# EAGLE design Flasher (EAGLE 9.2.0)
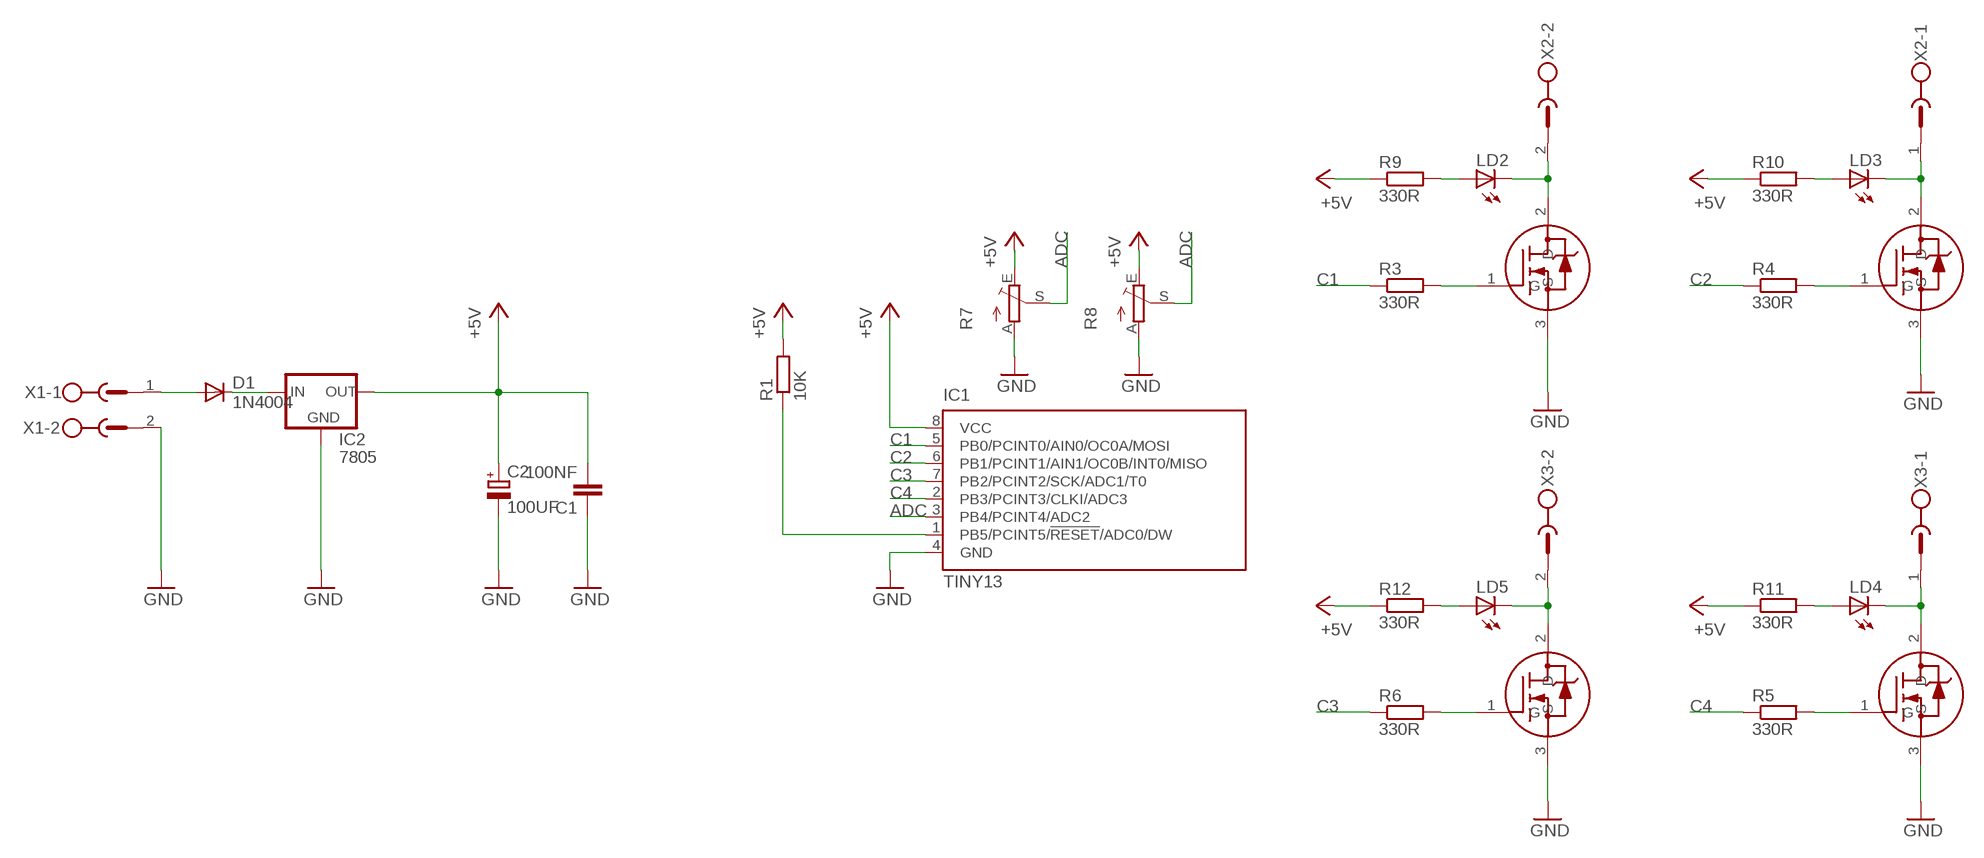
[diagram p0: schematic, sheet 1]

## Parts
C1  100NF  C-EU050-024X044  [C050-024X044]
C2  100UF  CPOL-EUE2.5-5  [E2,5-5]
D1  1N4004  [DO41-10]
IC1  TINY13  TINY13-20PU  [DIL08]
IC2  7805  78XXS  [78XXS]
LD2  LED5MM  [LED5MM]
LD3  LED5MM  [LED5MM]
LD4  LED5MM  [LED5MM]
LD5  LED5MM  [LED5MM]
R1  10K  R-EU_0204/7  [0204/7]
R3  330R  R-EU_0207/10  [0207/10]
R4  330R  R-EU_0207/10  [0207/10]
R5  330R  R-EU_0207/12  [0207/12]
R6  330R  R-EU_0207/10  [0207/10]
R7  TRIM_EU-B25U  [B25U]
R8  TRIM_EU-B25P  [B25P]
R9  330R  R-EU_0204/2V  [0204V]
R10  330R  R-EU_0204/2V  [0204V]
R11  330R  R-EU_0204/2V  [0204V]
R12  330R  R-EU_0204/2V  [0204V]
U$1  20N03  [DPAK]
U$2  20N03  [DPAK]
U$3  20N03  [DPAK]
U$4  20N03  [DPAK]
X1  MSTBV2  [MSTBV2]
X2  MSTBV2  [MSTBV2]
X3  MSTBV2  [MSTBV2]

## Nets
+5V: C1.2 C2.+ IC1.8(VCC) IC2.OUT R1.2 R7.E R8.E R9.1 R10.1 R11.1 R12.1
ADC: IC1.3(PB4/PCINT4/ADC2) R7.S R8.S
C1: IC1.5(PB0/PCINT0/AIN0/OC0A/MOSI) R3.1
C2: IC1.6(PB1/PCINT1/AIN1/OC0B/INT0/MISO) R4.1
C3: IC1.7(PB2/PCINT2/SCK/ADC1/T0) R6.1
C4: IC1.2(PB3/PCINT3/CLKI/ADC3) R5.1
GND: C1.1 C2.- IC1.4(GND) IC2.GND R7.A R8.A U$1.3(S) U$2.3(S) U$3.3(S) U$4.3(S) X1.2
N$1: LD2.K(C) U$1.2(D) X2.2
N$2: D1.A X1.1
N$3: D1.C IC2.IN
N$5: IC1.1(PB5/PCINT5/!RESET!/ADC0/DW) R1.1
N$6: LD3.K(C) U$3.2(D) X2.1
N$8: LD4.K(C) U$4.2(D) X3.1
N$9: R3.2 U$1.1(G)
N$10: R6.2 U$2.1(G)
N$11: R5.2 U$4.1(G)
N$12: R4.2 U$3.1(G)
N$13: LD2.A R9.2
N$14: LD3.A R10.2
N$15: LD4.A R11.2
N$16: LD5.A R12.2
N$17: LD5.K(C) U$2.2(D) X3.2

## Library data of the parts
C1 = rcl:C-EU: CAPACITOR, European symbol
C2 = rcl:CPOL-EU: POLARIZED CAPACITOR, European symbol
D1 = diode:1N4004: DIODE
IC1 = atmel:TINY13: 8-bit AVR Microcontroller with 1K Bytes In-System Programmable Flash Source: http://www.atmel.com/dyn/resources/prod_documents/2535S.pdf; MPN: ATTINY13-20PU; OC_FARNELL: 9171550; OC_NEWARK: 96K6521
IC2 = v-reg:78XXS: VOLTAGE REGULATOR
LD2-LD5 = led:LED: LED
R1 R3-R6 R9-R12 = rcl:R-EU_: RESISTOR, European symbol
R7 R8 = pot:TRIM_EU-: POTENTIOMETER
U$1-U$4 = 20n03:20N03
X1-X3 = con-phoenix-500:MSTBV2: PHOENIX; OC_FARNELL: unknown; OC_NEWARK: unknown

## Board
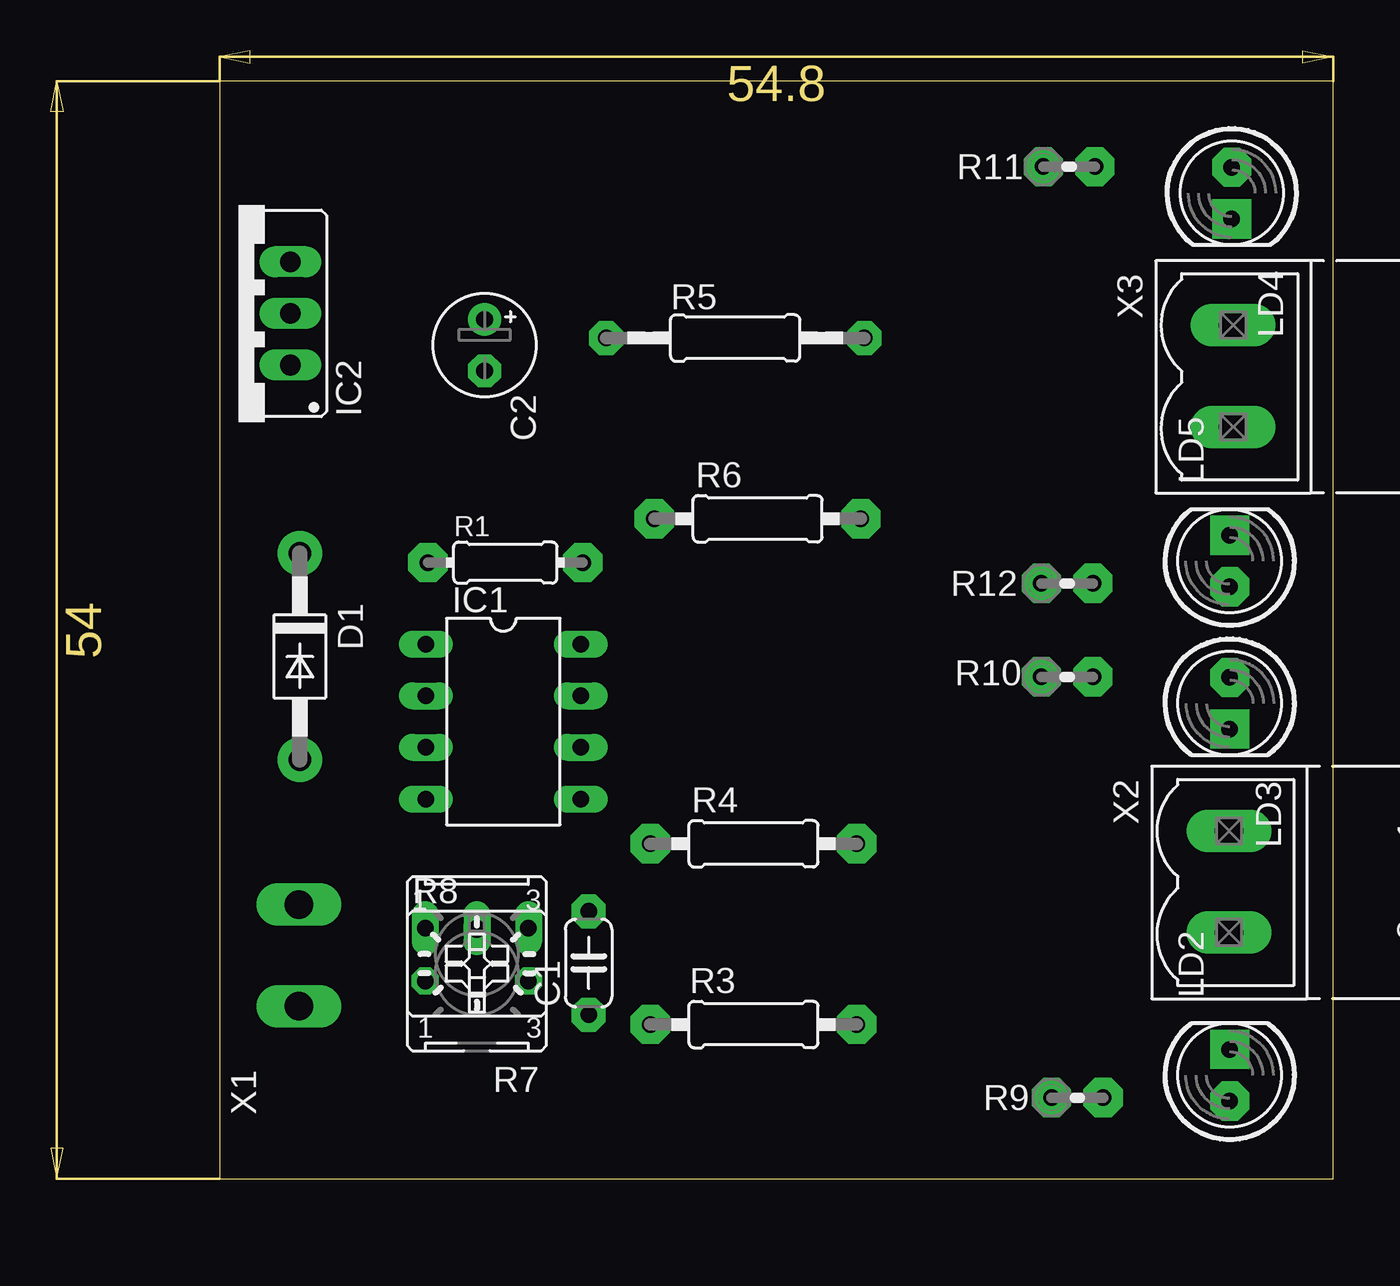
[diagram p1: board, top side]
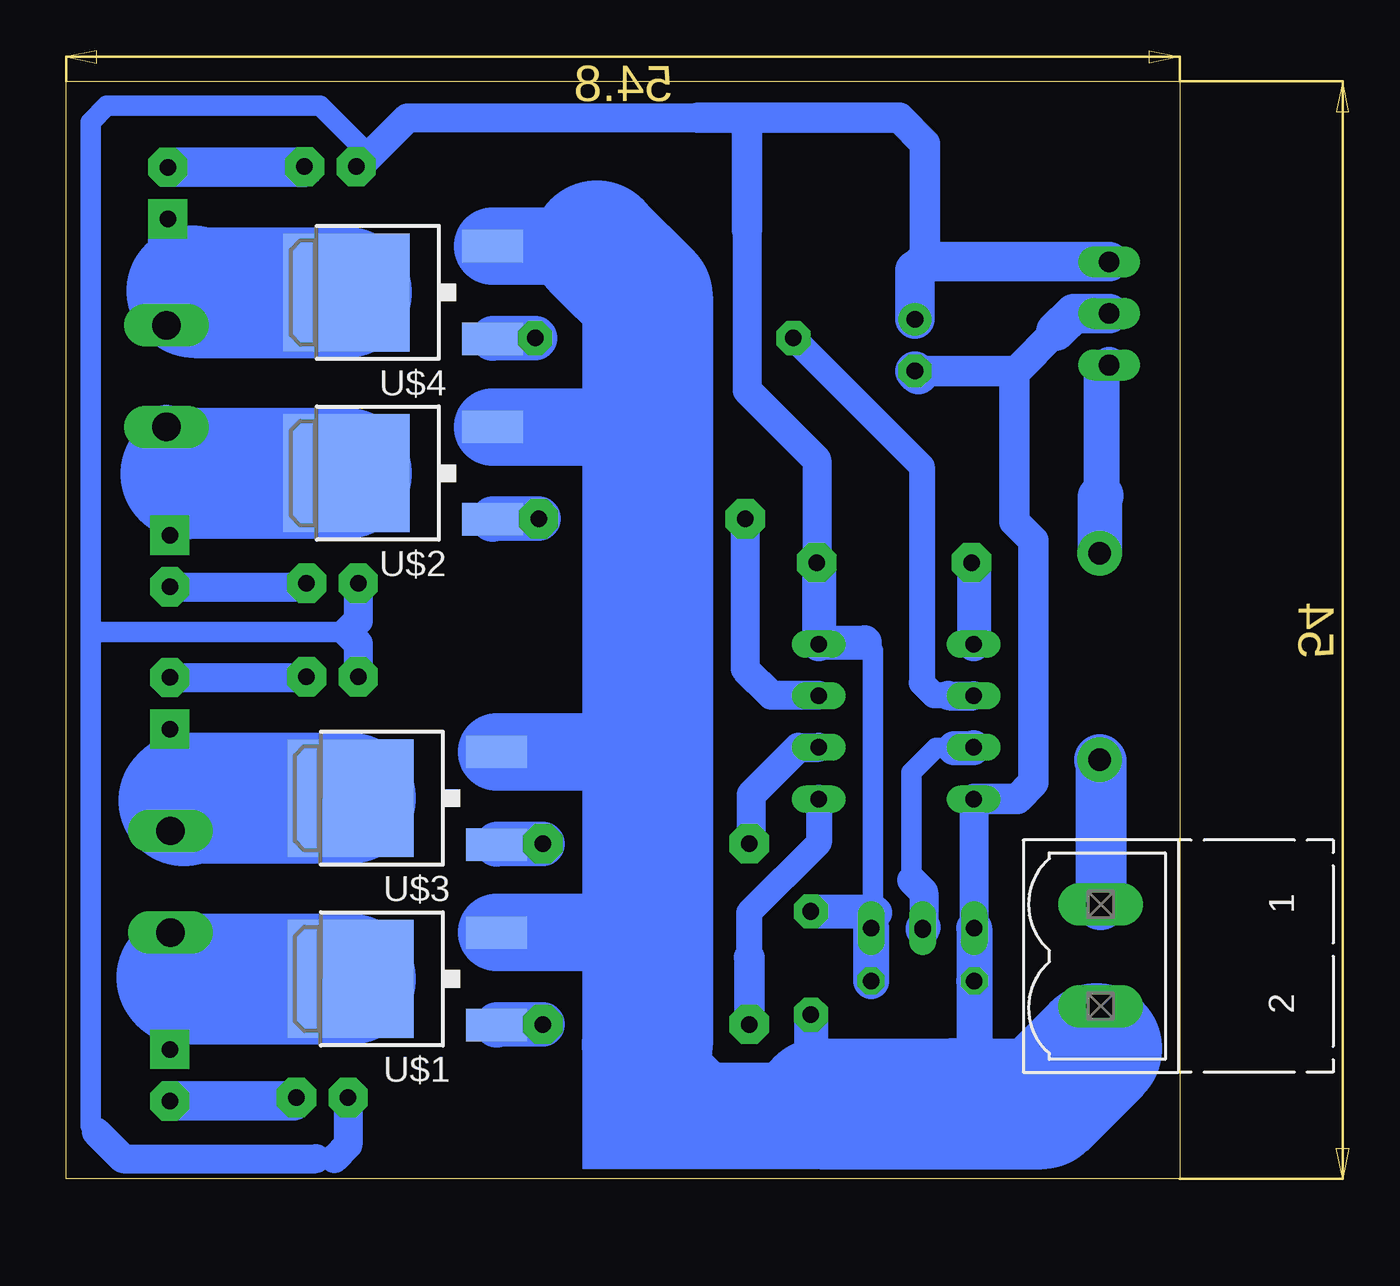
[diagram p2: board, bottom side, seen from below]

Size 63.1 x 55.5 mm. Coordinates in mm from the lower left corner, seen from the top.
Outline: 8.3,0 63.1,0 63.1,54 8.3,54 8.3,0
Copper layers (1*16): Top 0.035mm / dielectric 1.5mm / Bottom 0.035mm
Design rules "default": minimum track width 10mil, minimum drill 24mil, track to track 8mil, track to pad 8mil, pad to pad 8mil, via to via 8mil, smd to smd 8mil, copper to edge 40mil, drill to drill 8mil, minimum pad ring 10mil, minimum via ring 8mil, stop-mask expansion 4mil, vias tented up to drill 0mil, thermal gap 10mil

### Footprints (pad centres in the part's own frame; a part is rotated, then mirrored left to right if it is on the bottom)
C050-024X044 = drill 0.813 pad 1.676 octagon: 1 -2.54,0; 2 2.54,0
E2,5-5 = drill 0.813 pad 1.6: + -1.27,0 | drill 0.813 pad 1.6 octagon: - 1.27,0
DO41-10 = drill 1.118 pad 2.184: A 5.08,0; C -5.08,0
DIL08 = drill 0.813 long: 1 -3.81,-3.81; 2 -1.27,-3.81; 3 1.27,-3.81; 4 3.81,-3.81; 5 3.81,3.81; 6 1.27,3.81; 7 -1.27,3.81; 8 -3.81,3.81
78XXS = drill 1.016 long: GND 0,-2.54; IN -2.54,-2.54; OUT 2.54,-2.54
LED5MM = drill 0.813 pad 1.93 octagon: A -1.27,0 | drill 0.813 pad 1.93 square: K 1.27,0
0204/7 = drill 0.813 pad 1.93 octagon: 1 -3.81,0; 2 3.81,0
0207/10 = drill 0.813 pad 1.93 octagon: 1 -5.08,0; 2 5.08,0
0207/12 = drill 0.813 pad 1.676 octagon: 1 -6.35,0; 2 6.35,0
B25U = drill 0.813 long: A 2.54,-0.889; E -2.54,-0.889; S 0,-0.889
B25P = drill 0.813 octagon: A -2.54,0; E 2.54,0; S 0,2.54
0204V = drill 0.813 pad 1.93 octagon: 1 -1.27,0; 2 1.27,0
DPAK = smd 1.6 x 3: 1 -2.28,-4.8; 3 2.28,-4.8 | smd 5.8 x 6.2: 2 0,2.38
MSTBV2 = drill 1.397 long: 1 -2.5,0; 2 2.5,0

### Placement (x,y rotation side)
C1  26.46,10.62 90 top
C2  21.34,41.02 270 top
D1  12.25,25.7 270 top
IC1  22.26,22.5 270 top
IC2  9.24,42.58 90 top
LD2  58,5.1 90 top
LD3  58,23.4 270 top
LD4  58.1,48.5 270 top
LD5  58,30.4 90 top
R1  22.36,30.32 0 top
R3  34.57,7.6 0 top
R4  34.57,16.49 0 top
R5  33.67,41.37 0 top
R6  34.77,32.48 0 top
R7  20.96,11.44 180 top
R8  20.96,9.73 0 top
R9  50.5,4 0 top
R10  50,24.7 0 top
R11  50.1,49.8 0 top
R12  50,29.3 0 top
U$1  46.73,9.84 90 bottom
U$2  46.93,34.72 90 bottom
U$3  46.73,18.73 90 bottom
U$4  46.93,43.61 90 bottom
X1  12.2,11 270 bottom
X2  57.97,14.62 270 top
X3  58.17,39.5 270 top

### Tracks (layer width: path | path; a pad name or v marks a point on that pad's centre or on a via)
+5V
  Bottom 1.016: 61.6,2.3 61.9,2.6 61.9,26.9 | 61.9,26.9 61.9,52 61.1,52.8 50.6,52.8 48.7,50.9 48.7,49.93 R11.1 | 61.9,26.9 49.3,26.9 | 23.3,13.1 23.3,12 23.5,11.8 | 23.4,13.16 23.4,26 23.8,26.4
  Bottom 1.422: R11.1 48.7,49.8 46.3,52.2 32,52.2 | R9.1 49.23,1.67 49.9,1 | 50.8,1 60.3,1 61.6,2.3 | R12.1 48.73,27.47 49.3,26.9 48.73,26.33 R10.1 | R1.2 26.17,35.37 29.6,38.8 29.6,46.7
  Bottom 1.5: 29.6,52.2 22.1,52.2 20.84,50.94 20.84,45.12 | 32,52.2 29.6,52.2 | 29.6,52.2 29.6,46.7
  Bottom 1.676: 23.8,26.4 25.98,26.4 IC1.8 26.07,30.22 R1.2 | 21.34,44.7 21.3,44.66 | C1.2 23.4,13.16 | 23.36,13.16 23.3,13.1
  Bottom 1.778: R8.E 23.5,11.8 R7.E
  Bottom 1.93: IC2.OUT 20.84,45.12 21.3,44.66 | 21.34,44.7 C2.+
ADC
  Bottom 1.016: 19.4,21.2 20.3,21.2 21.5,20 21.5,14.7
  Bottom 1.422: 20.9,12.39 20.9,14.1 21.5,14.7
  Bottom 1.676: 19.4,21.2 18.48,21.2 IC1.3 | 20.9,12.39 R7.S R8.S
C1
  Bottom 1.27: 29.5,10.9 29.5,13.1 26.07,16.53 IC1.5
  Bottom 1.422: IC1.5 26.07,18.33 | R3.1 29.4,7.69
  Bottom 1.5: R3.1 29.49,10.89 29.5,10.9
C2
  Bottom 1.016: R4.1 29.4,16.58
  Bottom 1.422: IC1.6 27.07,21.23 29.4,18.9 29.4,16.58
C3
  Bottom 1.016: 26.1,23.8 IC1.7
  Bottom 1.422: R6.1 29.69,25.09 28.4,23.8 26.1,23.8
C4
  Bottom 1.27: 19.7,23.8 20.4,23.8 21,24.4 21,35.05 R5.1
  Bottom 1.422: IC1.2 19.67,23.77 19.7,23.8
GND
  Bottom 1.422: 34.5,43.4 33.1,44.8 | IC1.4 18.45,12.36 R7.A
  Bottom 1.5: C2.- 16.45,39.75 | 16.45,39.75 16.35,39.75 14.4,41.7 | 12.4,6.4 12.4,8.3 X1.2 | 16.45,39.75 16.45,32.35 15.5,31.4 15.5,19.5 16.31,18.69 IC1.4
  Bottom 1.676: C1.1 26.46,3.76 26.4,3.7
  Bottom 1.778: R7.A R8.A 18.42,3.72 18.4,3.7 | 19.42,3.72 19.4,3.7
  Bottom 1.93: 14.4,41.7 13.52,42.58 IC2.GND | C2.- 21.17,39.58
  Bottom 3.81: 37,45.9 U$4.3 | U$2.3 34.6,37 34.5,36.9 | U$3.3 35.11,21.01 35,20.9 34.5,20.9 | U$1.3 34.58,12.12 34.5,12.2 | 34,6.6 34.5,6.6 31.6,3.7 26.4,3.7 26,3.7
  Bottom 6.452: 12.4,6.4 15.1,3.7 18.4,3.7 19.4,3.7 26,3.7 | 34.5,6.6 34.5,12.2 34.5,20.9 34.5,36.9 34.5,43.4 37,45.9
N$1
  Bottom 1.93: 57.4,9.9 57.4,11.55 X2.2 | LD2.K 58,9.18 57.34,9.84
  Bottom 6.452: U$1.2 57.34,9.84 57.4,9.9
N$2
  Bottom 2.5: 12.2,20.57 X1.1
  Bottom 2.54: D1.A 12.2,20.57
N$3
  Bottom 1.778: IC2.IN 12.18,39.64 12.18,33.62
  Bottom 2.184: D1.C 12.25,33.55 12.18,33.62
N$5
  Bottom 1.676: IC1.1 18.45,30.22 R1.1
N$6
  Bottom 1.778: 57.3,18.6 57.3,18.3 57.3,17.79 X2.1
  Bottom 1.93: LD3.K 58,19 57.3,18.3
  Bottom 6.452: U$3.2 57.17,18.73 57.3,18.6
N$8
  Bottom 1.93: LD4.K 58.1,44.9 56.9,43.7
  Bottom 2.184: 56.9,43.7 56.9,43.27 X3.1
  Bottom 6.452: U$4.2 56.81,43.61 56.9,43.7
N$9
  Bottom 2.184: R3.2 41.89,7.6 U$1.1
N$10
  Bottom 2.184: R6.2 42.09,32.48 U$2.1
N$11
  Bottom 2.184: R5.2 42.09,41.37 U$4.1
N$12
  Bottom 2.184: R4.2 41.89,16.49 U$3.1
N$13
  Bottom 1.93: LD2.A 51.94,3.83 R9.2
N$14
  Bottom 1.422: LD3.A 51.3,24.67 R10.2
N$15
  Bottom 1.93: LD4.A 51.4,49.77 R11.2
N$16
  Bottom 1.422: LD5.A 51.44,29.13 R12.2
N$17
  Bottom 1.93: 58,33.9 LD5.K
  Bottom 2.184: X3.2 57.2,36.03 57.2,34.7 58,33.9
  Bottom 6.452: U$2.2 57.18,34.72 57.2,34.7
(copper drawn outside any net)
  shapes: Bottom area x2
